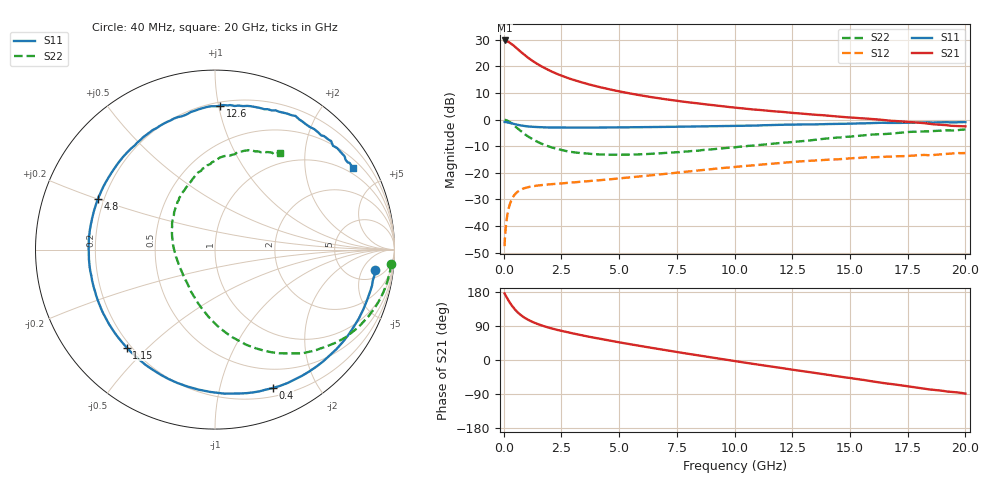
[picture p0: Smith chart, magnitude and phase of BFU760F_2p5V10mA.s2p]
! Filename:  P:\Prog\Test\Noise\ATS_data\Testdata_Net\Split files Spar\BFU760F_2W_C1_Bias3_2.5V_5mA_30mA_D.s2p
! Date/Time: Mon 06/Feb/2012 15:08:07
! BFU760_2W_C1_Bias3_2.5V_5mA_30mA_R.s2p
! MDIF S-parameter v. bias file
! BFU760_2W_C1_2.5V_5mA_30mA
! Date/time Fri Mar 18 11:16:19 2011
! VAR V_out= 2.5000
! VAR I_out= 10.0800
! VAR V_in= 0.7711
! VAR I_in= 0.0279
! Device data file deembeded for feedlines and parallel
! Original file: \Split files Spar\BFU760_2W_C1_Bias3_2.5V_5mA_30mA_R.s2p
! Feed-files: PR003V01_101208_Feed1.s2p, PR003V01_101208_Feed2.s2p
! Parallel-file: PR003V01_101208_Par.s2p
# MHz S MA R 50
!  Freq-MHz  S11-mag  S11-arg  S21-mag  S21-arg  S12-mag  S12-arg  S22-mag  S22-arg
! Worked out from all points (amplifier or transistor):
!   167 points, 40 MHz to 20 GHz, reference 50 ohm
!   highest |S21| = 29.7 dB at 40 MHz (marker M1)
!   |S21| within 3 dB of that: start of sweep to 574.4 MHz
!   unconditionally stable (mu >= 1): 5.197 GHz to 12.78 GHz; 12.87 GHz to 13.06 GHz
!   at 550 MHz: K = 0.14, MSG = 27.2 dB, |S12| = -27.5 dB
!   at 4.2 GHz: K = 0.89, MSG = 17.4 dB, |S12| = -22.8 dB
!   at 20 GHz: K = 0.83, MSG = 5.0 dB, |S12| = -12.6 dB
!   S11 on the Smith chart (normalised r, x): 40 MHz: 8, -9; 400 MHz: 0.29, -1.46; 1.15 GHz: 0.18, -0.43; 4.8 GHz: 0.18, +0.20; 12.6 GHz: 0.23, +1.01; 20 GHz: 0.78, +3.49
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40  0.8987 -7.4  30.48 175.4  0.004187 77.6  0.9843 -4.6
50  0.8993 -9.4  30.45 173.8  0.005703 76.5  0.983 -5.9
140  0.8886 -25.5  29.59 164.2  0.01439 75.0  0.9606 -16.6
240  0.8694 -42.9  28.12 153.8  0.0235 67.1  0.9119 -27.6
320  0.8541 -55.4  26.49 146.6  0.02967 61.1  0.8622 -35.8
400  0.8355 -67.4  25.05 139.8  0.03482 55.9  0.8073 -42.9
550  0.8042 -86.2  22.05 129.1  0.04199 47.6  0.7088 -54.7
650  0.7855 -96.7  20.14 123.3  0.04556 43.3  0.6526 -61.2
750  0.7718 -105.9  18.5 118.2  0.04829 39.8  0.6006 -66.9
950  0.7503 -120.6  15.69 109.9  0.05218 34.5  0.5161 -76.4
1150  0.7349 -132.0  13.51 103.3  0.05481 30.8  0.4524 -84.3
1500  0.7196 -146.8  10.77 94.4  0.0578 26.8  0.3742 -95.8
1950  0.708 -160.1  8.463 85.4  0.06045 24.0  0.3126 -107.6
2500  0.705 -171.9  6.66 76.9  0.06315 22.6  0.2684 -120.1
3400  0.7048 173.8  4.952 65.1  0.06791 21.7  0.2339 -136.2
4800  0.7108 156.5  3.517 48.9  0.07685 21.6  0.2189 -158.3
6800  0.7248 136.7  2.478 28.1  0.09342 19.6  0.2324 175.6
10200  0.7651 107.4  1.642 -4.7  0.1307 9.0  0.3078 137.7
12600  0.8014 88.0  1.32 -26.4  0.1602 -2.8  0.3809 115.2
13400  0.8076 82.3  1.238 -33.4  0.1698 -8.0  0.4114 107.8
16800  0.8639 55.7  0.946 -63.5  0.2016 -28.8  0.5433 78.2
20000  0.8933 30.6  0.7436 -88.6  0.2343 -50.9  0.6482 55.8
